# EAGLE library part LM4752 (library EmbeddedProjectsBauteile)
National Semiconductor Stereo 11W Audio Power Amplifier
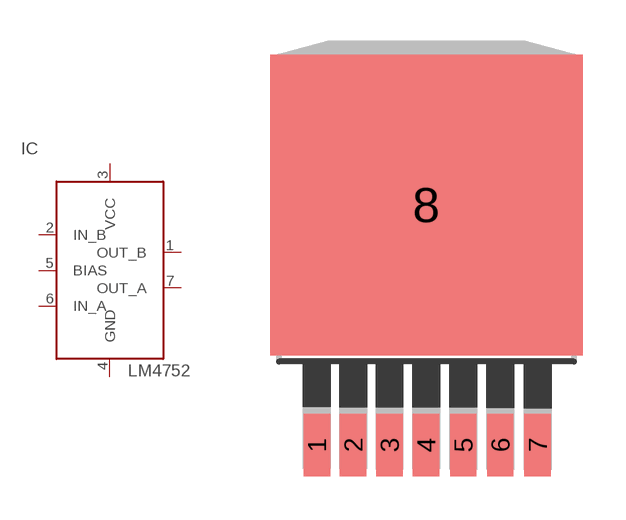
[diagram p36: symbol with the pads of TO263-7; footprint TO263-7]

Designator prefix IC

## LM4752TS (EP: 400222)  [TO263-7]
1  OUT_B  out
2  IN_B  in
3  VCC  pwr
4  GND  pwr
5  BIAS  in
6  IN_A  in
7  OUT_A  out

## Footprint TO263-7 (pad centres in mm)
smd 0.914 x 2.159: 1 -3.794,-8.311; 2 -2.535,-8.311; 3 -1.278,-8.311; 4 -0.014,-8.311; 5 1.271,-8.311; 6 2.552,-8.311; 7 3.847,-8.311
smd 10.8 x 10.41: 8 0,0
